(* Logix 5000 AddOnInstructionDefinition export CM1T_ControlMode; software revision 20.00 *)

TYPE CM1T_DriveStatus :
STRUCT
   StatusValue : SINT;   // Indicates status and error type
   StatusValue1 : SINT;   // Additional status values
   In_Position : BOOL;   // Drive is in position and ready to move
   Moving : BOOL;   // Drive is currently moving
   Disabled : BOOL;   // Drive is disabled
   Error : BOOL;   // Drive is in an error state
   MoveComplete : BOOL;   // Move Complete
   NewStartRequired : BOOL;   // New setpoint required
   HomeAchieved : BOOL;   // Home achieved
END_STRUCT
END_TYPE

TYPE CM1T_Controlword :
STRUCT
   Start : BOOL;   // Start a motion or set a new setpoint
   Halt : BOOL;   // Halt the current motion
   Relative_Move : BOOL;   // Execute the position profile as a relative move
   Speed_Control : BOOL;   // Execute the profile as speed control only
   Disable : BOOL;   // Disable the drive (zero torque)
   Reset_Error : BOOL;   // Reset any existing errors with rising edge
   Set_to_Zero : BOOL;   // Set the current position to 0
   Home : BOOL;   // Execute a home search
END_STRUCT
END_TYPE

TYPE CM1T_Axis :
STRUCT
   Input : SINT[32];   // Data coming from the CM1-T
   Output : SINT[20];   // Data going to the CM1-T
   us50Counter : DINT;   // Controller 50us counter
   ClearCounter : BOOL;
   ModeOfOperation : SINT;   // Type of motion control mode
   ModeOfOperationDisplay : SINT;   // Indicates the active control mode
   Controlword : CM1T_Controlword;   // Controls the drive operation
   DriveStatus : CM1T_DriveStatus;   // Shows status of the drive
   PositionTarget : DINT;   // Final target position for position move
   SpeedTarget : DINT;   // Maximum speed for target move
   TorqueTarget : INT;   // Max torque allowed in 0.1% of peak. Typically 1100
   AccelerationTarget : INT;   // Acceleration for profile move
   DecelerationTarget : INT;   // Deceleration for profile move
   PositionActual : DINT;   // Actual position of the drive
   TargetActual : DINT;   // 1ms position target
   PositionError : DINT;   // Error between the current drive position and the instantaneous target position
   SpeedActual : DINT;   // Actual speed of the drive
   CurrentActual : INT;   // 0.1% of rated current
   OverloadActual : INT;   // 0.1% of overload torque
   DCVoltage : INT;   // DC voltage bus. 0.1V unit
   AnalogIN : INT;   // Value of 10bit analog input
   DigitalIN : SINT;   // Read the digital inputs
   DigitalOUT : SINT;   // Set the digital outputs
   Temperature : SINT;   // Temperature of the drive
   ErrorCode : SINT;   // Indicates error in Ethernet/IP module
END_STRUCT
END_TYPE

ADD_ON_INSTRUCTION CM1T_ControlMode   (* revision 1.0 *)
// Control Mode
VAR_INPUT
   ControlMode_Value : DINT; {required}
END_VAR
VAR_IN_OUT
   CM1T_Axis : CM1T_Axis; {required}
END_VAR

ROUTINE Logic   (* ladder *)
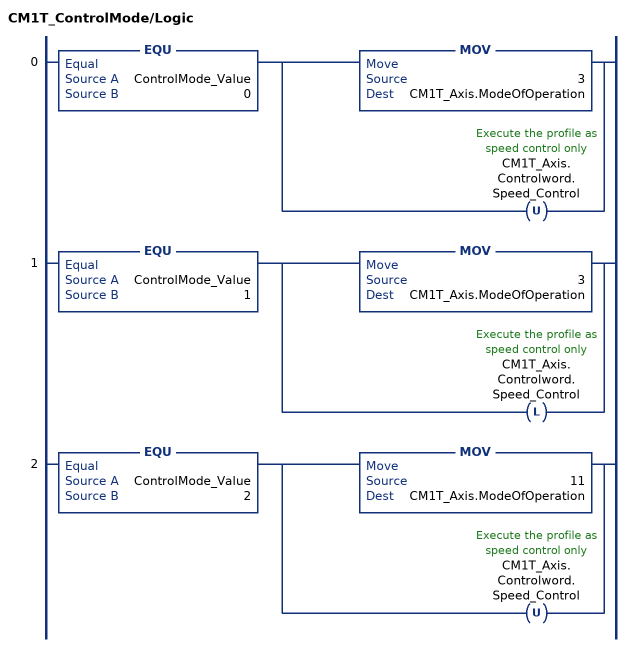
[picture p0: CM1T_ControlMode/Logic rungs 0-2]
   0: EQU(ControlMode_Value,0)[MOV(3,CM1T_Axis.ModeOfOperation) ,OTU(CM1T_Axis.Controlword.Speed_Control) ];
   1: EQU(ControlMode_Value,1)[MOV(3,CM1T_Axis.ModeOfOperation) ,OTL(CM1T_Axis.Controlword.Speed_Control) ];
   2: EQU(ControlMode_Value,2)[MOV(11,CM1T_Axis.ModeOfOperation) ,OTU(CM1T_Axis.Controlword.Speed_Control) ];
END_ROUTINE
END_ADD_ON_INSTRUCTION
